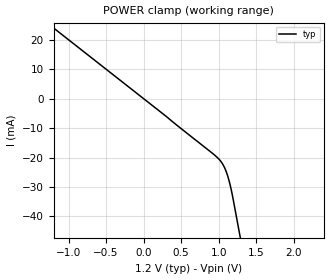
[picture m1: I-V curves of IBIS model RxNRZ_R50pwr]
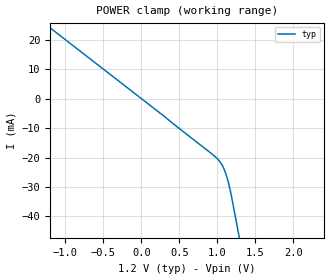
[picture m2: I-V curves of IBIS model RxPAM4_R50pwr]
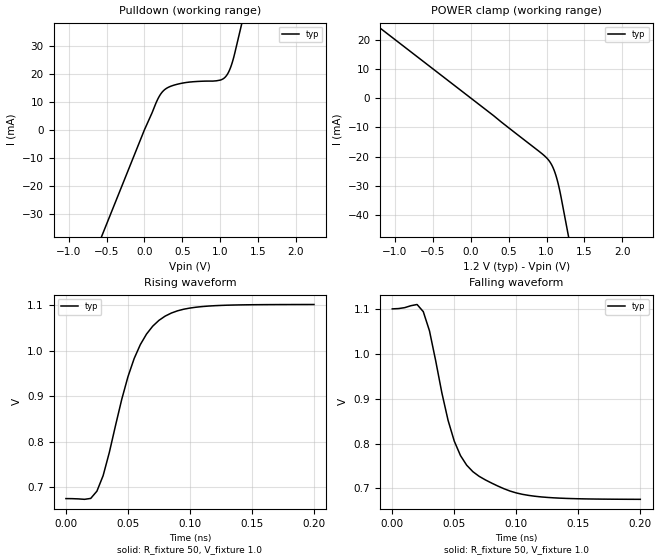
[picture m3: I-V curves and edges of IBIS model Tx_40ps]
[IBIS Ver]   5.1
[Disclaimer] THESE IBIS MODELS ARE PROVIDED "AS IS" WITH NO
   WARRANTY WHATSOEVER AND Mentor Graphics Inc.
   SPECIFICALLY DISCLAIMS ANY IMPLIED WARRANTIES OF
   MERCHANTABILITY, FITNESS FOR A PARTICULAR PURPOSE,
   OR AGAINST INFRINGEMENT.
[File Name]  generic_serdes_wpkg.ibs
[File Rev]   0.3
[Date]   6/20/2018
[Source]   Developed by:  Mentor Graphics Inc.
[Notes]   This IBIS file uses a HyperLynx proprietary syntax
   to use the Touschtone package model.  Consequently
   this file will only parse without errors with the
   HyperLynx IBIS Parser.
[Copyright] Copyright 2010, Mentor Graphics, Inc.,
   All Rights Reserved.
[Component]   Generic_SERDES
[Manufacturer] None
[Package]
R_pkg   0.0   NA   NA
L_pkg   0.0   NA   NA
C_pkg   0.0   NA   NA
[Pin]   signal_name   model_name   R_pin  L_pin  C_pin
1p   TxP   Tx   NA   NA   NA
1n   TxN   Tx   NA   NA   NA
2p   RxP   Rx   NA   NA   NA
2n   RxN   Rx   NA   NA   NA
3p   RxP_PAM4   Rx_PAM4   NA   NA   NA
3n   RxN_PAM4   Rx_PAM4   NA   NA   NA
[Diff Pin] inv_pin  vdiff  tdelay_typ  tdelay_min  tdelay_max
1p   1n   0.1V   NA   NA   NA
2p   2n   0.1V   NA   NA   NA
3p   3n   0.1V   NA   NA   NA
|************************** DIE NODES ***************************
[Node Declarations]
1p_die
1n_die
2p_die
2n_die
3p_die
3n_die
[End Node Declarations]
|*** CIRCUIT CALLS to insert node between buffer out and pin ****
[Circuit Call] Tx
Port_map A_signal 1p_die
Signal_pin 1p
[End Circuit Call]
[Circuit Call] Tx
Port_map A_signal 1n_die
Signal_pin 1n
[End Circuit Call]
[Circuit Call] Rx
Port_map A_signal 2p_die
Signal_pin 2p
[End Circuit Call]
[Circuit Call] Rx
Port_map A_signal 2n_die
Signal_pin 2n
[End Circuit Call]
[Circuit Call] Rx_PAM4
Port_map A_signal 3p_die
Signal_pin 3p
[End Circuit Call]
[Circuit Call] Rx_PAM4
Port_map A_signal 3n_die
Signal_pin 3n
[End Circuit Call]
|*********** CIRCUIT CALLS to connect package models ************
[Circuit Call]  pkg_model_20180620_s4p
Port_map 1 1p_die
Port_map 2 1p
Port_map 3 1n_die
Port_map 4 1n
[End Circuit Call]
[Circuit Call]  pkg_model_20180620_s4p
Port_map 1 2p_die
Port_map 2 2p
Port_map 3 2n_die
Port_map 4 2n
[End Circuit Call]
[Circuit Call]  pkg_model_20180620_s4p
Port_map 1 3p_die
Port_map 2 3p
Port_map 3 3n_die
Port_map 4 3n
[End Circuit Call]
[Model Selector] Tx
Tx_40ps   Driver with an approximately 40ps edge
Tx_20ps   Driver with an approximately 20ps edge
Tx_10ps   Driver with an approximately 10ps edge
Tx_5ps   Driver with an approximately 5ps edge
Tx_2p5ps   Driver with an approximately 2.5ps edge
[Model Selector] Rx
RxNRZ   Receiver with NRZ AMI model, no ODT
RxNRZ_R50pwr   Receiver with NRZ AMI model, 50 Ohm ODT to POWER
[Model Selector] Rx_PAM4
RxPAM4   Receiver with PAM4 AMI model, no ODT
RxPAM4_R50pwr   Receiver with PAM4 AMI model, 50 Ohm ODT to POWER
|******************** EXTERNAL CIRCUIT CALLS ********************
[External Circuit]  pkg_model_20180620_s4p
Language SPICE
Corner  Typ  .\pkg_model_20180620_s4p.sp  pkg_model_20180620_s4p
Ports 1 2 3 4
[End External Circuit]
[Model]   RxNRZ
Model_type  Input
C_comp 0.00p 0.00p 0.00p
Vinh = 0.55
Vinl = 0.45
[Temperature_Range]  25   100   0
[Voltage Range]   1.2   1.14  1.26
[Algorithmic Model]
Executable   Windows_VisualStudio_32   MentorRx_32.dll   MentorRx.ami
Executable   Windows_VisualStudio_64   MentorRx_64.dll   MentorRx.ami
Executable   Linux_gcc3.2.3_32   libMentorRx_32.so   MentorRx.ami
Executable   Linux_gcc3.2.3_64   libMentorRx_64.so   MentorRx.ami
[End Algorithmic Model]
[Model]   RxPAM4
Model_type  Input
C_comp 0.00p 0.00p 0.00p
Vinh = 0.55
Vinl = 0.45
[Temperature_Range]  25   100   0
[Voltage Range]   1.2   1.14  1.26
[Algorithmic Model]
Executable   Windows_VisualStudio_32   MentorRxPAM4_32.dll   MentorRxPAM4.ami
Executable   Windows_VisualStudio_64   MentorRxPAM4_64.dll   MentorRxPAM4.ami
Executable   Linux_gcc3.2.3_32   libMentorRxPAM4_32.so  MentorRxPAM4.ami
Executable   Linux_gcc3.2.3_64   libMentorRxPAM4_64.so  MentorRxPAM4.ami
[End Algorithmic Model]
| Models and submodels in the file (9): RxNRZ (Input), RxNRZ_R50pwr (Input), RxPAM4 (Input), RxPAM4_R50pwr (Input), Tx_40ps (Open_sink), Tx_20ps (Open_sink), Tx_10ps (Open_sink), Tx_5ps (Open_sink), Tx_2p5ps (Open_sink)
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[Model]   RxNRZ_R50pwr
Model_type  Input
C_comp 0.00p 0.00p 0.00p
Vinh = 0.55
Vinl = 0.45
[Temperature_Range]  25   100   0
[Voltage Range]   1.2   1.14  1.26
[POWER Clamp]
-1.2V     24mA       NA         NA
300mV     -6mA       NA         NA
975mV     -19.81mA   NA         NA
1.05V     -22.08mA   NA         NA
1.1V      -24.74mA   NA         NA
1.13V     -27.08mA   NA         NA
1.15V     -29mA      NA         NA
1.17V     -31.22mA   NA         NA
1.2V      -35.12mA   NA         NA
2.4V      -199.3mA   NA         NA
[Algorithmic Model]
Executable   Windows_VisualStudio_32   MentorRx_32.dll   MentorRx.ami
Executable   Windows_VisualStudio_64   MentorRx_64.dll   MentorRx.ami
Executable   Linux_gcc3.2.3_32   libMentorRx_32.so   MentorRx.ami
Executable   Linux_gcc3.2.3_64   libMentorRx_64.so   MentorRx.ami
[End Algorithmic Model]
[Model]   RxPAM4_R50pwr
Model_type  Input
C_comp 0.00p 0.00p 0.00p
Vinh = 0.55
Vinl = 0.45
[Temperature_Range]  25   100   0
[Voltage Range]   1.2   1.14  1.26
[POWER Clamp]
-1.2V     24mA       NA         NA
300mV     -6mA       NA         NA
975mV     -19.81mA   NA         NA
1.05V     -22.08mA   NA         NA
1.1V      -24.74mA   NA         NA
1.13V     -27.08mA   NA         NA
1.15V     -29mA      NA         NA
1.17V     -31.22mA   NA         NA
1.2V      -35.12mA   NA         NA
2.4V      -199.3mA   NA         NA
[Algorithmic Model]
Executable   Windows_VisualStudio_32   MentorRxPAM4_32.dll   MentorRxPAM4.ami
Executable   Windows_VisualStudio_64   MentorRxPAM4_64.dll   MentorRxPAM4.ami
Executable   Linux_gcc3.2.3_32   libMentorRxPAM4_32.so  MentorRxPAM4.ami
Executable   Linux_gcc3.2.3_64   libMentorRxPAM4_64.so  MentorRxPAM4.ami
[End Algorithmic Model]
[Model]   Tx_40ps
Model_type  Open_sink
C_comp 1.0p  NA  NA
Cref = 0
Vref = 0.8
Rref = 50
Vmeas = 0.8
[Temperature_Range]  25   100   0
[Voltage Range]   1.2   1.14  1.26
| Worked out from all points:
|   slope of the pulldown table from 0 to 0.18 V, typ, clamps not added: 16.1 ohm
|   falling waveform, R_fixture 50, V_fixture 1.0: 20-80 % time 25.2ps typ, NA min, NA max; typ from 1.1 V to 0.675 V
|   rising waveform, R_fixture 50, V_fixture 1.0: 20-80 % time 27.2ps typ, NA min, NA max; typ from 0.675 V to 1.1 V
[Pulldown]
-1.2V     -80.86mA   NA         NA
0V        0A         NA         NA
180mV     11.16mA    NA         NA
270mV     14.38mA    NA         NA
360mV     15.65mA    NA         NA
520mV     16.73mA    NA         NA
1.01V     17.8mA     NA         NA
1.06V     18.63mA    NA         NA
1.11V     20.57mA    NA         NA
1.16V     24.13mA    NA         NA
1.2V      28.29mA    NA         NA
2.4V      165.4mA    NA         NA
[POWER Clamp]
-1.2V     24mA       NA         NA
300mV     -6mA       NA         NA
975mV     -19.81mA   NA         NA
1.05V     -22.08mA   NA         NA
1.1V      -24.74mA   NA         NA
1.13V     -27.08mA   NA         NA
1.15V     -29mA      NA         NA
1.17V     -31.22mA   NA         NA
1.2V      -35.12mA   NA         NA
2.4V      -199.3mA   NA         NA
[Ramp]
| variable   typ   min   max
dV/dt_r   0.256/2.719E-11   NA   NA
dV/dt_f   0.256/2.525E-11   NA   NA
R_load = 50ohms
[Falling Waveform]
R_fixture = 50
V_fixture = 1.0
| Time   V(typ)   V(min)  V(max)
0s        1.101V     NA         NA
20ps      1.111V     NA         NA
25ps      1.095V     NA         NA
30ps      1.052V     NA         NA
40ps      913.1mV    NA         NA
50ps      805.2mV    NA         NA
55ps      773mV      NA         NA
65ps      737mV      NA         NA
110ps     683.9mV    NA         NA
200ps     675.1mV    NA         NA
[Rising Waveform]
R_fixture = 50
V_fixture = 1.0
| Time   V(typ)   V(min)  V(max)
0s        674.9mV    NA         NA
20ps      675.4mV    NA         NA
25ps      691.3mV    NA         NA
30ps      725.4mV    NA         NA
45ps      892.7mV    NA         NA
55ps      982.3mV    NA         NA
65ps      1.036V     NA         NA
75ps      1.066V     NA         NA
110ps     1.097V     NA         NA
200ps     1.101V     NA         NA
[Algorithmic Model]
Executable   Windows_VisualStudio_32   MentorTx_32.dll   MentorTx.ami
Executable   Windows_VisualStudio_64   MentorTx_64.dll   MentorTx.ami
Executable   Linux_gcc3.2.3_32   libMentorTx_32.so   MentorTx.ami
Executable   Linux_gcc3.2.3_64   libMentorTx_64.so   MentorTx.ami
[End Algorithmic Model]
